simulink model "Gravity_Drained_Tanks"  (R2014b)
settings: Solver=ode45  StartTime=0.0  StopTime=500  RelTol=1e-3
PreLoadFcn:
  | Initialize
StopFcn:
  | Plot_and_save
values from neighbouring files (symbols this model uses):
  P = P    (= 0)    [mpc.m]
undefined symbols (not defined in the file or in its folder): PlotTanks
libraries: simulink x2

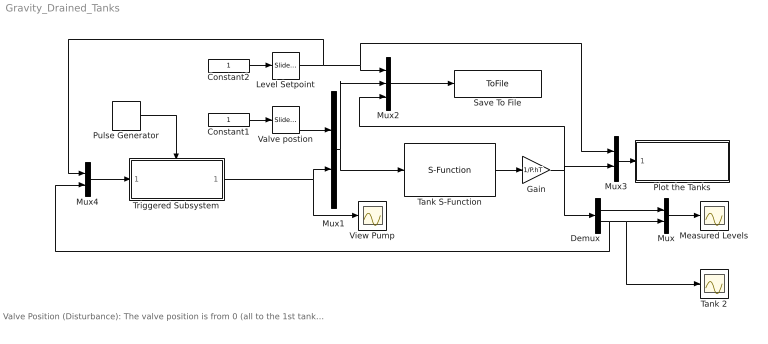
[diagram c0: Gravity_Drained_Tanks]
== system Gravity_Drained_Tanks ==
  note: Valve Position (Disturbance): The valve position is from 0 (all to the 1st tank) to 1 (all to the 2nd) Pump Output (MV): The output is from 0 to 1 which corresponds to a fraction of the maximum flow rate. Change blue box values (slider).
  Constant1 : Constant
  Constant2 : Constant
  Demux : Demux  Outputs=2
  Gain : Gain  Gain=1/P.hT
  Level Setpoint : simulink/Math Operations/Slider Gain  low=0  gain=0.5  high=1
  Measured Levels : Scope
  Mux{,1,3..4} (4 alike) : Mux  Inputs=2
  Mux2 : Mux  Inputs=3
  Plot the Tanks : Subsystem
  Pulse Generator : DiscretePulseGenerator  PulseType=Time based  Period=1  PulseWidth=5
  Save To File : ToFile  Filename=data_manual.mat  MatrixName=tanks  SampleTime=1
  Tank 2 : Scope
  Tank S-Function : S-Function  FunctionName=tank_dynamics  Parameters=P  EnableBusSupport=off
  Triggered Subsystem : Subsystem  TreatAsAtomicUnit=on
  Valve postion : simulink/Math Operations/Slider Gain  low=0  gain=0  high=1
  View Pump : Scope
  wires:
  Gain/1 -> Mux3/2, Demux/1, Mux2/3
  Tank S-Function/1 -> Gain/1
  Mux2/1 -> Save To File/1
  Constant1/1 -> Valve postion/1
  Mux1/1 -> Mux2/2, Tank S-Function/1
  Triggered Subsystem/1(Out1) -> View Pump/1, Mux1/2
  Valve postion/1 -> Mux1/1
  Constant2/1 -> Level Setpoint/1
  Level Setpoint/1 -> Mux4/1, Mux3/1, Mux2/1
  Mux3/1 -> Plot the Tanks/1(h)
  Mux/1 -> Measured Levels/1
  Demux/1 -> Mux/1
  Demux/2 -> Mux4/2, Tank 2/1, Mux/2
  Mux4/1 -> Triggered Subsystem/1(In1)
  Pulse Generator/1 -> Triggered Subsystem/Trigger

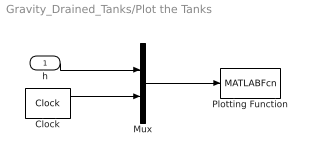
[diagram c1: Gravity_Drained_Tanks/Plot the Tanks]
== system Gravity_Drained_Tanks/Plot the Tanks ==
  h : Inport
  Clock : Clock
  Mux : Mux  Inputs=2
  Plotting Function : MATLABFcn  MATLABFcn=PlotTanks(u)  OutputDimensions=0  SampleTime=.2
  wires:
  Mux/1 -> Plotting Function/1
  Clock/1 -> Mux/2
  h/1 -> Mux/1

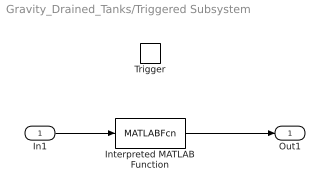
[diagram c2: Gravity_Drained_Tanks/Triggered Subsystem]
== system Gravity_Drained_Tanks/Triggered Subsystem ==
  In1 : Inport
  Trigger : TriggerPort
  Interpreted MATLAB Function : MATLABFcn  MATLABFcn=mpc
  Out1 : Outport  InitialOutput=[0]
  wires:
  In1/1 -> Interpreted MATLAB Function/1
  Interpreted MATLAB Function/1 -> Out1/1
